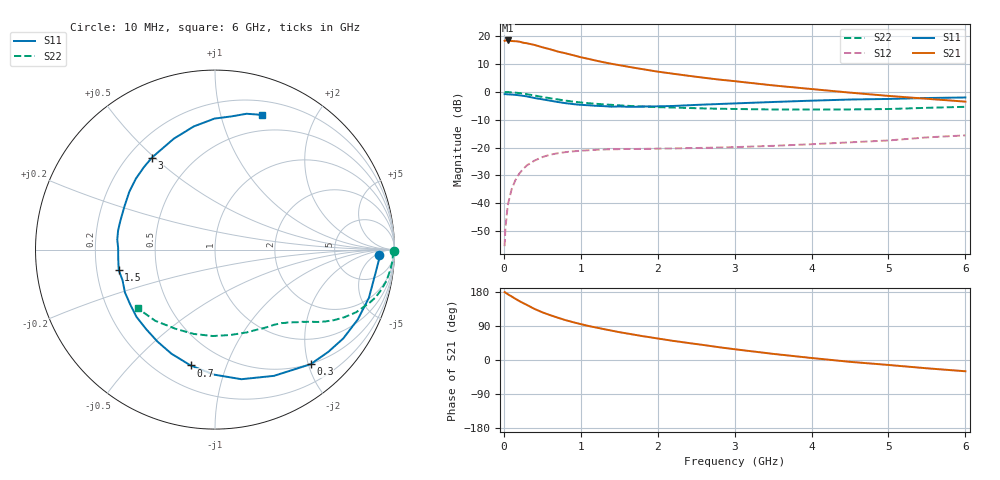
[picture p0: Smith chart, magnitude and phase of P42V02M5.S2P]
! SIEMENS Small Signal Semiconductors
! BFP182
! Si NPN RF Bipolar Junction Transistor in SOT143
! VCE = 2 V  IC = 2.5 mA
! Common Emitter S-Parameters:  March  1996
# GHz  S  MA  R  50
!  f  S11  S21  S12  S22
! GHz  MAG  ANG  MAG  ANG  MAG  ANG  MAG  ANG
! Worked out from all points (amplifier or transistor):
!   36 points, 10 MHz to 6 GHz, reference 50 ohm
!   highest |S21| = 18.5 dB at 50 MHz (marker M1)
!   |S21| within 3 dB of that: start of sweep to 578.4 MHz
!   unconditionally stable (mu >= 1): 2.005 GHz to 5.918 GHz
!   at 250 MHz: K = 0.14, MSG = 22.7 dB, |S12| = -27.7 dB
!   at 1.4 GHz: K = 0.74, MSG = 15.3 dB, |S12| = -20.6 dB
!   at 6 GHz: K = 0.99, MSG = 6.1 dB, |S12| = -15.6 dB
!   S11 on the Smith chart (normalised r, x): 10 MHz: 19, -7; 300 MHz: 0.49, -2.04; 700 MHz: 0.33, -0.76; 1.5 GHz: 0.29, -0.10; 3 GHz: 0.29, +0.49; 6 GHz: 0.33, +1.35
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0.01  0.9127 -1.9  8.261 179.1  0.0017 82.1  0.9958 -0.6
0.02  0.915 -3.6  8.378 178.1  0.0035 88.1  0.9905 -1.3
0.05  0.9029 -8.9  8.392 173.8  0.0091 88.0  0.992 -3.5
0.1  0.8986 -17.4  8.196 167.8  0.0177 79.5  0.9818 -7.0
0.2  0.8694 -34.7  7.992 155.7  0.034 70.2  0.9534 -13.5
0.3  0.8315 -50.2  7.462 145.3  0.048 62.2  0.9104 -19.0
0.4  0.7762 -65.0  6.968 134.6  0.0586 54.7  0.8609 -23.9
0.5  0.7369 -78.5  6.338 125.9  0.0675 48.0  0.8122 -27.7
0.6  0.6965 -90.5  5.836 118.5  0.0745 43.1  0.7715 -30.6
0.7  0.6596 -101.9  5.314 111.7  0.0792 39.0  0.7331 -33.1
0.8  0.6288 -112.7  4.941 105.3  0.0829 35.2  0.6995 -35.2
0.9  0.6043 -122.1  4.568 99.8  0.0857 32.3  0.6697 -36.9
1.1  0.5759 -139.5  3.92 89.8  0.0896 27.4  0.6274 -39.9
1.3  0.5555 -154.7  3.402 81.5  0.0927 23.7  0.5978 -42.6
1.5  0.5483 -168.0  3.022 73.5  0.0938 21.4  0.5734 -45.1
1.8  0.5474 174.1  2.568 63.1  0.0949 19.5  0.5461 -49.0
2.2  0.5591 154.5  2.121 50.5  0.0966 18.0  0.5239 -54.9
3  0.6217 124.4  1.56 28.4  0.102 17.8  0.4938 -69.2
3.5  0.6591 110.4  1.309 16.2  0.1076 18.3  0.4835 -79.6
4.5  0.73 90.2  0.971 -4.8  0.1243 18.7  0.4845 -104.1
5.5  0.7771 76.9  0.753 -21.9  0.1526 17.3  0.5181 -130.1
6  0.7948 70.8  0.669 -29.7  0.166 13.9  0.5404 -142.7
